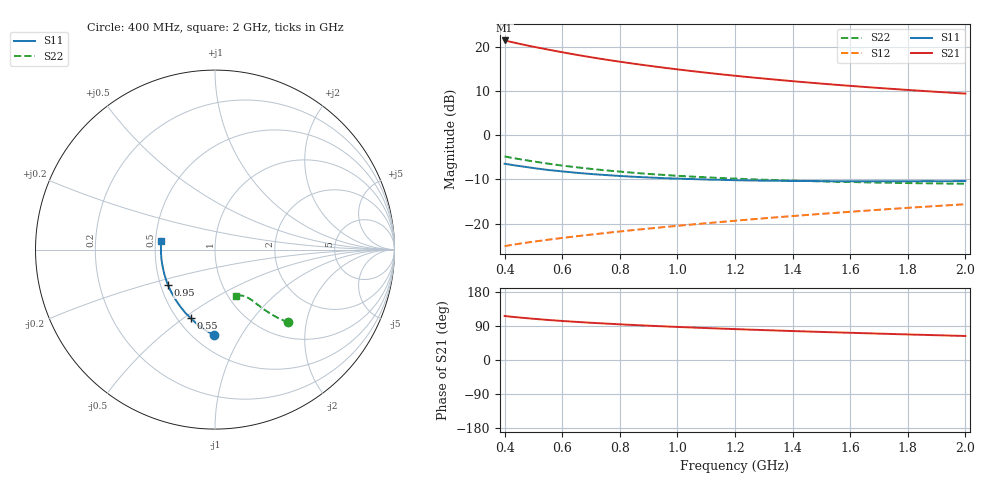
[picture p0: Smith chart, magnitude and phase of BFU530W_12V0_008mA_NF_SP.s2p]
! Filename:  P:\Prog\Test\Noise\ATS_data\Testdata_Net\06 Compressed Noise after Statistics\BFU530W_APM2013_09_A05_12p0V_008mA_NF_CM01_D.sf
! Date/Time: Tue 26/Mar/2013 18:06:01
! BFU530W_APM2013_09_A05_12p0V_1to25mA_NF_CM01_Bias5_R.sf
! Noise Parameter Data File
! BFU530W_APM2013_09_A05_12p0V_1to25mA_NF_CM01
! Date/time: Thu Mar 21 22:54:15 2013
! VAR V_out= 12.000000
! VAR I_out= 8.005000
! VAR V_in= 0.800100
! VAR I_in= 0.069810
! Device data file deembeded for feedlines and parallel
! Original file: \06 Compressed Noise after Statistics\BFU530W_APM2013_09_A05_12p0V_008mA_NF_CM01_R.sf
! Feed-files: PR019V01_070313_Feed1.s2p, PR019V01_070313_Feed2.s2p
! Parallel-file: PR019V01_070313_Par.s2p
# MHz S MA R 50
!  Freq-MHz  S11-mag  S11-arg  S21-mag  S21-arg  S12-mag  S12-arg  S22-mag  S22-arg
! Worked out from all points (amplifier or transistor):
!   37 points, 400 MHz to 2 GHz, reference 50 ohm
!   highest |S21| = 21.4 dB at 400 MHz (marker M1)
!   |S21| within 3 dB of that: start of sweep to 628.9 MHz
!   unconditionally stable (mu >= 1): 1.563 GHz to end of sweep
!   at 500 MHz: K = 0.64, MSG = 22.0 dB, |S12| = -24.1 dB
!   at 1.1 GHz: K = 0.93, MSG = 17.0 dB, |S12| = -19.9 dB
!   at 2 GHz: K = 1.02, MAG = 11.7 dB, |S12| = -15.6 dB
!   lowest NFmin = 0.74 dB at 420 MHz
!   S11 on the Smith chart (normalised r, x): 400 MHz: 0.62, -0.77; 550 MHz: 0.58, -0.53; 950 MHz: 0.55, -0.24; 2 GHz: 0.54, +0.06
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400  0.4759 -90.8  11.74 116.1  0.05574 57.8  0.5744 -44.7
420  0.4642 -93.6  11.35 114.5  0.05726 57.5  0.559 -45.5
440  0.4533 -96.4  10.97 112.9  0.05864 57.3  0.5441 -46.2
460  0.4439 -98.9  10.62 111.5  0.06 57.2  0.5307 -46.8
480  0.4346 -101.5  10.29 110.2  0.06134 57.1  0.5176 -47.3
500  0.4253 -104.0  9.969 108.8  0.06263 57.0  0.5048 -47.8
550  0.4047 -109.5  9.268 105.7  0.06582 57.1  0.4772 -48.9
600  0.3899 -114.9  8.638 103.0  0.06905 57.2  0.4532 -49.8
650  0.376 -119.6  8.078 100.6  0.07218 57.4  0.4337 -50.6
700  0.3641 -124.3  7.586 98.2  0.07531 57.7  0.416 -51.3
750  0.3548 -128.5  7.145 96.2  0.07845 58.0  0.4003 -51.7
800  0.3457 -132.5  6.753 94.2  0.08169 58.4  0.3879 -52.4
850  0.3387 -136.3  6.402 92.3  0.08487 58.7  0.3752 -52.8
950  0.3272 -143.1  5.796 88.9  0.09133 59.5  0.356 -53.6
1050  0.3193 -149.2  5.294 85.8  0.09789 60.1  0.3405 -54.5
1150  0.313 -155.0  4.871 82.9  0.1046 60.6  0.3277 -55.3
1200  0.3099 -157.5  4.689 81.5  0.1081 60.8  0.3233 -55.9
1350  0.3051 -164.7  4.21 77.7  0.1185 61.4  0.3104 -57.2
1500  0.3023 -171.2  3.822 74.0  0.1291 61.7  0.3007 -59.0
1650  0.3007 -177.2  3.504 70.7  0.1399 61.9  0.2933 -60.7
1750  0.3011 179.3  3.324 68.5  0.1474 61.9  0.2899 -61.9
2000  0.3039 171.0  2.946 63.4  0.166 61.6  0.2832 -65.5
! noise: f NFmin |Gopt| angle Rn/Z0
400  0.751  0.0483  67.82  0.0963
460  0.7442  0.05654  74.82  0.0966
600  0.7622  0.07727  73.92  0.1024
800  0.7977  0.07214  96.19  0.0981
1000  0.8123  0.1083  117.5  0.0925
1200  0.8531  0.1211  127.5  0.0927
1400  0.8921  0.1484  144.5  0.0849
1600  0.911  0.1707  151.9  0.0777
1800  0.9289  0.1757  167.7  0.0845
2000  0.9757  0.1884  -179.4  0.0849
